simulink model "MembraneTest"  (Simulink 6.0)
settings: Solver=ode45  StartTime=0.0  StopTime=SimTime  FixedStep=0.001  RelTol=1e-3
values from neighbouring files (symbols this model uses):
  A0 = 0    [ScriptFour.m]    (also in SinPureTest.m)
  A1 = 0    [ScriptFour.m]
  A2 = 0    [ScriptFour.m]
  A3 = 0    [ScriptFour.m]
  A4 = 0    [ScriptFour.m]
  A5 = 0    [ScriptFour.m]
  b = S/Sm    (= 0.1)    [Constantes.m]    (also in ConstantesBck.m)
  B1 = 1    [ScriptFour.m]
  B2 = 1/3    (= 0.333333333333)    [ScriptFour.m]
  B3 = 1/5    (= 0.2)    [ScriptFour.m]
  B4 = 1/7    (= 0.142857142857)    [ScriptFour.m]
  B5 = 1/9    (= 0.111111111111)    [ScriptFour.m]
  C = 1    [Constantes.m]    (also in ConstantesBck.m)
  Fact = 10^2    (= 100)    [Constantes.m]    (also in ConstantesBck.m)
  FreqStim = 1/(2*pi*i)    (= 0.318309886184)    [ScriptFour.m]    (also in HalfSin.m = 1/(2*pi*i); SinPureTest.m = 1/(2*pi*i); SinPureTestFreq.m = 1/(2*pi*i))
  GainI = AddI    (= 0)    [ScriptFour.m]
  gk = 36    [Constantes.m]    (also in ConstantesBck.m; sim_hh.m)
  gl = 0.3    [Constantes.m]    (also in ConstantesBck.m; sim_hh.m)
  gna = 120    [Constantes.m]    (also in ConstantesBck.m; sim_hh.m)
  h0 = 0.5961    [Constantes.m]    (also in ConstantesBck.m)
  m0 = 0.0529    [Constantes.m]    (also in ConstantesBck.m)
  mK = 0    [Constantes.m]    (also in ConstantesBck.m)
  mL = 0    [Constantes.m]    (also in ConstantesBck.m)
  mNa = 0    [Constantes.m]    (also in ConstantesBck.m)
  n0 = 0.3177    [Constantes.m]    (also in ConstantesBck.m)
  PhaseStim = 0    [ScriptFour.m]    (also in SinPureTest.m; SinPureTestFreq.m)
  Sm = 3.14e-2    (= 0.0314)    [Constantes.m]    (also in ConstantesBck.m = 0.000314)
  Vk = -82    [Constantes.m]    (also in ConstantesBck.m)
  Vl = -59    [Constantes.m]    (also in ConstantesBck.m)
  Vna = 45    [Constantes.m]    (also in ConstantesBck.m)
  Vr = -70    [Constantes.m]    (also in ConstantesBck.m)

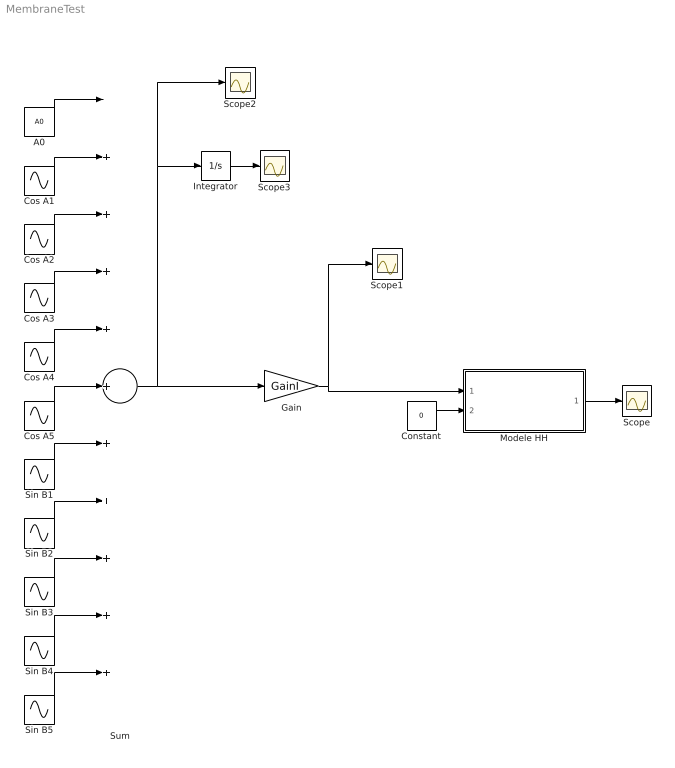
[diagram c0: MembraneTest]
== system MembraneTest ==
  A0 : Constant  Value=A0
  Constant : Constant  Value=0
  Cos A1 : Sin  Amplitude=A1  Frequency=FreqStim  Phase=PhaseStim+pi/2  SampleTime=0
  Cos A2 : Sin  Amplitude=A2  Frequency=3*FreqStim  Phase=PhaseStim+pi/2  SampleTime=0
  Cos A3 : Sin  Amplitude=A3  Frequency=5*FreqStim  Phase=PhaseStim+pi/2  SampleTime=0
  Cos A4 : Sin  Amplitude=A4  Frequency=7*FreqStim  Phase=PhaseStim+pi/2  SampleTime=0
  Cos A5 : Sin  Amplitude=A5  Frequency=9*FreqStim  Phase=PhaseStim+pi/2  SampleTime=0
  Gain : Gain  Gain=GainI
  Integrator : Integrator
  Modele HH : Subsystem
  Scope{,1..3} (4 alike) : Scope
  Sin B1 : Sin  Amplitude=B1  Frequency=FreqStim  Phase=PhaseStim  SampleTime=0
  Sin B2 : Sin  Amplitude=B2  Frequency=3*FreqStim  Phase=PhaseStim  SampleTime=0
  Sin B3 : Sin  Amplitude=B3  Frequency=5*FreqStim  Phase=PhaseStim  SampleTime=0
  Sin B4 : Sin  Amplitude=B4  Frequency=7*FreqStim  Phase=PhaseStim  SampleTime=0
  Sin B5 : Sin  Amplitude=B5  Frequency=9*FreqStim  Phase=PhaseStim  SampleTime=0
  Sum : Sum  Inputs=|+++++++++++
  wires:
  Modele HH/1(HHout) -> Scope/1
  Constant/1 -> Modele HH/2(VRefIn)
  Sin B5/1 -> Sum/11
  Sin B4/1 -> Sum/10
  Sin B3/1 -> Sum/9
  Sin B2/1 -> Sum/8
  Sin B1/1 -> Sum/7
  Cos A5/1 -> Sum/6
  Cos A4/1 -> Sum/5
  Cos A3/1 -> Sum/4
  Cos A2/1 -> Sum/3
  Cos A1/1 -> Sum/2
  A0/1 -> Sum/1
  Sum/1 -> Scope2/1, Integrator/1, Gain/1
  Gain/1 -> Modele HH/1(HHin), Scope1/1
  Integrator/1 -> Scope3/1

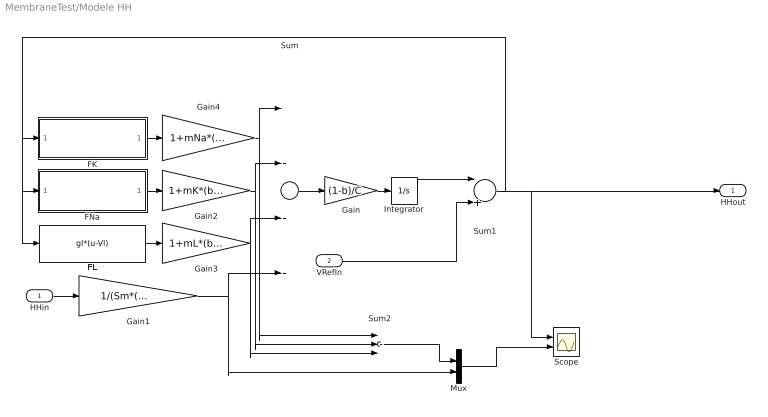
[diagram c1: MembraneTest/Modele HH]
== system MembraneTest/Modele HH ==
  HHin : Inport  Port=1  LatchInput=off
  VRefIn : Inport  Port=2  LatchInput=off
  FK : Subsystem
  FL : Fcn  Expr=gl*(u-Vl)
  FNa : Subsystem
  Gain : Gain  Gain=(1-b)/C
  Gain1 : Gain  Gain=1/(Sm*(1-b)*Fact)
  Gain2 : Gain  Gain=1+mK*(b/(1-b))
  Gain3 : Gain  Gain=1+mL*(b/(1-b))
  Gain4 : Gain  Gain=1+mNa*(b/(1-b))
  Integrator : Integrator  InitialCondition=Vr
  Mux : Mux  Inputs=2
  Scope : Scope  NumInputPorts=2
  Sum : Sum  Inputs=|---+
  Sum1 : Sum  Inputs=|++
  Sum2 : Sum  Inputs=|+++
  HHout : Outport
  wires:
  Sum/1 -> Gain/1
  Gain/1 -> Integrator/1
  FK/1(FKout) -> Gain4/1
  FNa/1(FNaOut) -> Gain2/1
  FL/1 -> Gain3/1
  HHin/1 -> Gain1/1
  Integrator/1 -> Sum1/1
  Sum1/1 -> FNa/1(FNaIn), FL/1, FK/1(FKIn), HHout/1, Scope/1
  Gain1/1 -> Sum/4, Mux/2
  Gain4/1 -> Sum/1, Sum2/1
  Gain2/1 -> Sum/2, Sum2/2
  Gain3/1 -> Sum/3, Sum2/3
  VRefIn/1 -> Sum1/2
  Sum2/1 -> Mux/1
  Mux/1 -> Scope/2

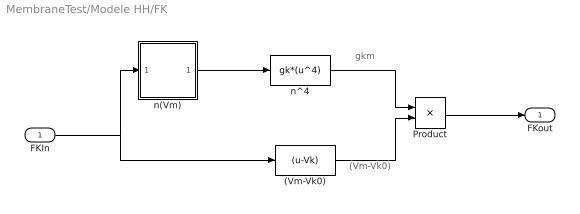
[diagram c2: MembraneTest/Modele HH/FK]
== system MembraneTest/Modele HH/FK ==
  note: gkm
  note: (Vm-Vk0)
  FKIn : Inport  Port=1  LatchInput=off
  (Vm-Vk0) : Fcn  Expr=(u-Vk)
  Product : Product
  n(Vm) : Subsystem
  n^4 : Fcn  Expr=gk*(u^4)
  FKout : Outport  InitialOutput=0
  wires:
  n(Vm)/1(n) -> n^4/1
  (Vm-Vk0)/1 -> Product/2
  Product/1 -> FKout/1
  n^4/1 -> Product/1
  FKIn/1 -> n(Vm)/1(Vm), (Vm-Vk0)/1

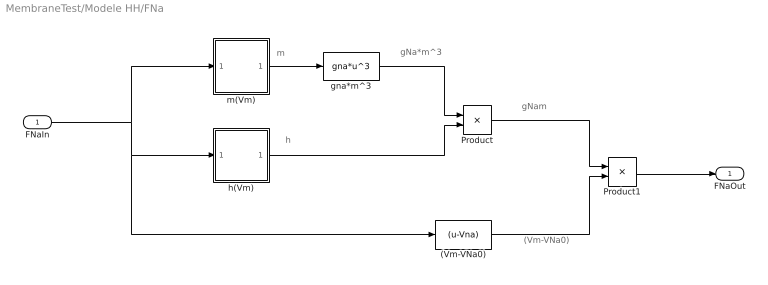
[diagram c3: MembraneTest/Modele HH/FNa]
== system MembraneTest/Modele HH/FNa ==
  note: gNa*m^3
  note: m
  note: h
  note: gNam
  note: (Vm-VNa0)
  FNaIn : Inport  Port=1  LatchInput=off
  (Vm-VNa0) : Fcn  Expr=(u-Vna)
  Product : Product
  Product1 : Product
  gna*m^3 : Fcn  Expr=gna*u^3
  h(Vm) : Subsystem
  m(Vm) : Subsystem
  FNaOut : Outport  InitialOutput=0
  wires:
  (Vm-VNa0)/1 -> Product1/2
  gna*m^3/1 -> Product/1
  Product1/1 -> FNaOut/1
  FNaIn/1 -> m(Vm)/1(Vm), h(Vm)/1(Vm), (Vm-VNa0)/1
  m(Vm)/1(n) -> gna*m^3/1
  h(Vm)/1(h) -> Product/2
  Product/1 -> Product1/1

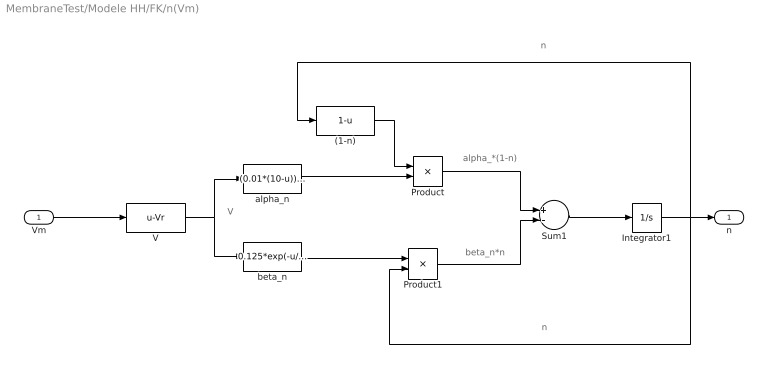
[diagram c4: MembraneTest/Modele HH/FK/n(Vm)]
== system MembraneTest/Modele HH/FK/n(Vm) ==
  note: V
  note: alpha_*(1-n)
  note: beta_n*n
  note: n
  note: n
  Vm : Inport  Port=1  LatchInput=off
  (1-n) : Fcn  Expr=1-u
  Integrator1 : Integrator  InitialCondition=n0
  Product : Product
  Product1 : Product
  Sum1 : Sum  Inputs=+-
  V : Fcn  Expr=u-Vr
  alpha_n : Fcn  Expr=(0.01*(10-u))/(exp((10-u)/10)-1)
  beta_n : Fcn  Expr=0.125*exp(-u/80)
  n : Outport  InitialOutput=0
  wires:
  V/1 -> alpha_n/1, beta_n/1
  alpha_n/1 -> Product/2
  (1-n)/1 -> Product/1
  beta_n/1 -> Product1/1
  Product/1 -> Sum1/1
  Product1/1 -> Sum1/2
  Sum1/1 -> Integrator1/1
  Integrator1/1 -> (1-n)/1, Product1/2, n/1
  Vm/1 -> V/1

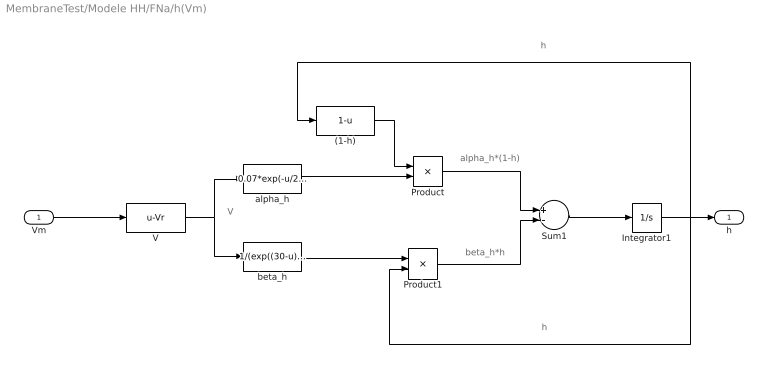
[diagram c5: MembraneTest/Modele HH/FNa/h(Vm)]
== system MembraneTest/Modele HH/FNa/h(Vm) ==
  note: h
  note: h
  note: beta_h*h
  note: alpha_h*(1-h)
  note: V
  Vm : Inport  Port=1  LatchInput=off
  (1-h) : Fcn  Expr=1-u
  Integrator1 : Integrator  InitialCondition=h0
  Product : Product
  Product1 : Product
  Sum1 : Sum  Inputs=+-
  V : Fcn  Expr=u-Vr
  alpha_h : Fcn  Expr=0.07*exp(-u/20)
  beta_h : Fcn  Expr=1/(exp((30-u)/10)+1)
  h : Outport  InitialOutput=0
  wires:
  Vm/1 -> V/1
  Integrator1/1 -> h/1, Product1/2, (1-h)/1
  Sum1/1 -> Integrator1/1
  Product1/1 -> Sum1/2
  Product/1 -> Sum1/1
  beta_h/1 -> Product1/1
  (1-h)/1 -> Product/1
  alpha_h/1 -> Product/2
  V/1 -> beta_h/1, alpha_h/1

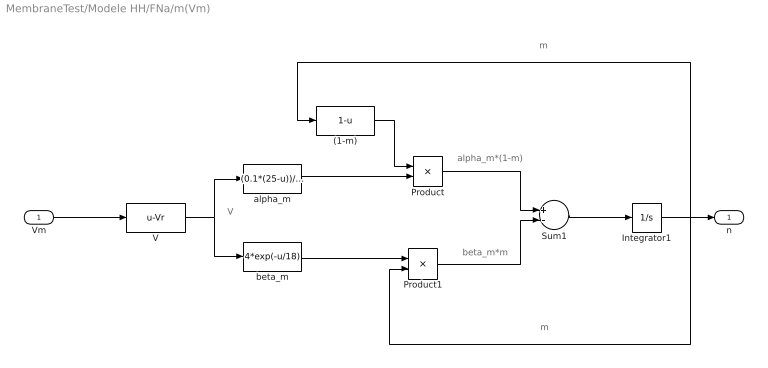
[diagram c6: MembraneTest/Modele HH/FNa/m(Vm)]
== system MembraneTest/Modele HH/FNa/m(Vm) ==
  note: m
  note: m
  note: beta_m*m
  note: alpha_m*(1-m)
  note: V
  Vm : Inport  Port=1  LatchInput=off
  (1-m) : Fcn  Expr=1-u
  Integrator1 : Integrator  InitialCondition=m0
  Product : Product
  Product1 : Product
  Sum1 : Sum  Inputs=+-
  V : Fcn  Expr=u-Vr
  alpha_m : Fcn  Expr=(0.1*(25-u))/(exp((25-u)/10)-1)
  beta_m : Fcn  Expr=4*exp(-u/18)
  n : Outport  InitialOutput=0
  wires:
  Vm/1 -> V/1
  Integrator1/1 -> n/1, Product1/2, (1-m)/1
  Sum1/1 -> Integrator1/1
  Product1/1 -> Sum1/2
  Product/1 -> Sum1/1
  beta_m/1 -> Product1/1
  (1-m)/1 -> Product/1
  alpha_m/1 -> Product/2
  V/1 -> beta_m/1, alpha_m/1
